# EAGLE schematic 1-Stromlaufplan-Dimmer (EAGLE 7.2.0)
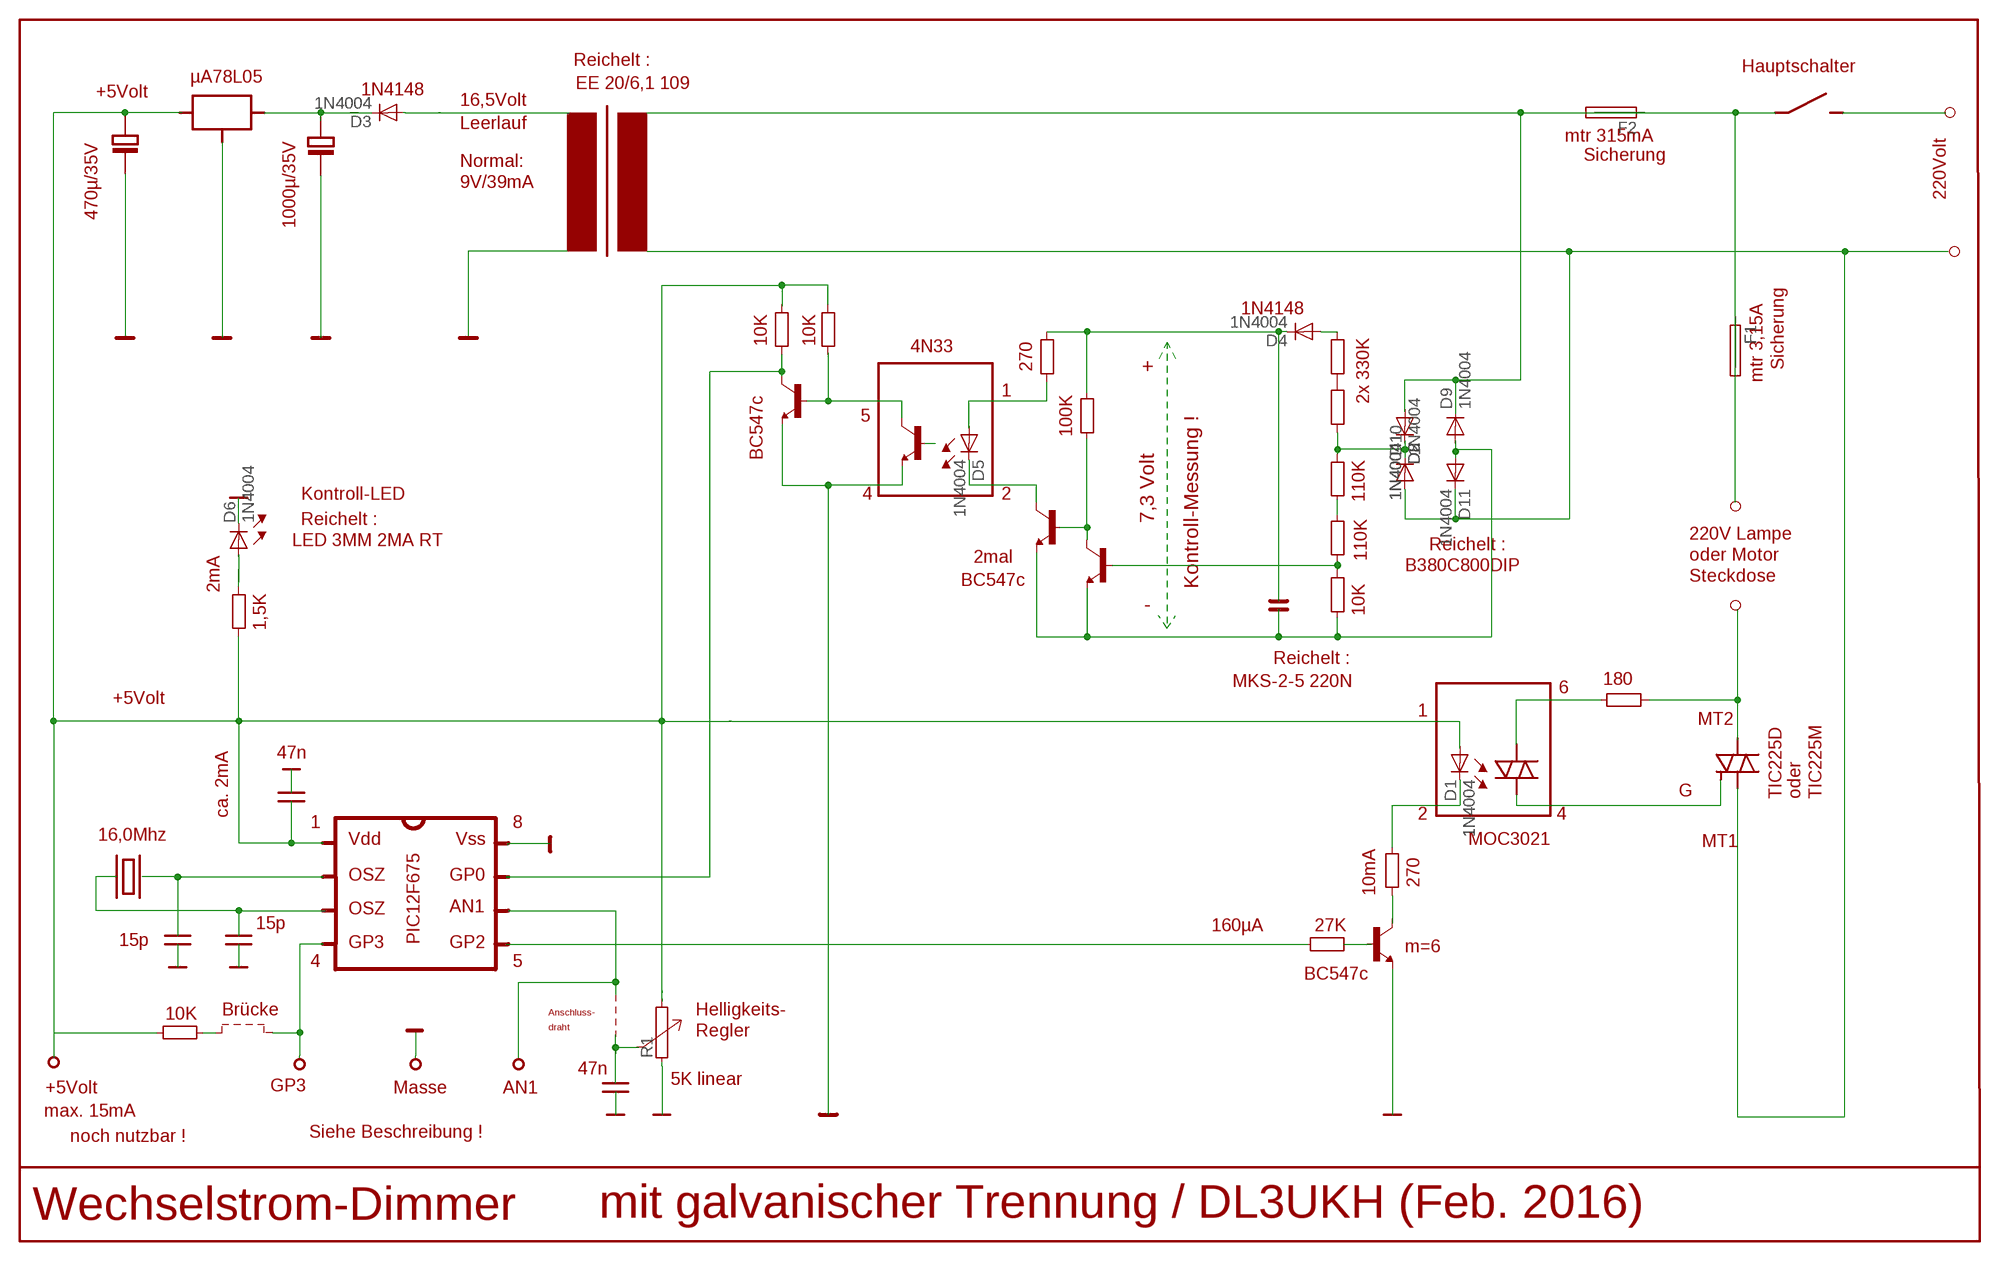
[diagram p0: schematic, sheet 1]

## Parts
D1  1N4004  [DO41-10]
D2  1N4004  [DO41-10]
D3  1N4004  [DO41-10]
D4  1N4004  [DO41-10]
D5  1N4004  [DO41-10]
D6  1N4004  [DO41-10]
D8  1N4004  [DO41-10]
D9  1N4004  [DO41-10]
D10  1N4004  [DO41-10]
D11  1N4004  [DO41-10]
F1  19559  [19559]
F2  19559  [19559]
R1  RHS10  [HS10]

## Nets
N$6: R1.1
N$23: D1.A R1.2
N$27: D1.C
N$28: D2.C D8.C D10.C
N$31: D3.A
N$35: D3.C
N$38: D4.A
N$39: D4.C
N$44: F1.1 F1.2
N$47: D2.A D8.A D9.C F2.1 F2.2
N$49: D9.A D11.A
N$50: D10.A D11.C
N$51: D5.A
N$56: D5.C
N$63: D6.A
N$64: D6.C

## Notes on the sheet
- Reichelt :
- Hauptschalter
- +5Volt | µA78L05
- EE 20/6,1 109
- 1N4148
- 16,5Volt
- Leerlauf
- mtr 315mA | 220Volt
- Sicherung
- Normal:
- 9V/39mA
- 470µ/35V
- 1000µ/35V
- Sicherung
- 1N4148
- 2x 330K
- 10K | 10K
- 4N33
- 270 | +
- mtr 3,15A
- 1
- 5
- 100K
- BC547c
- Kontroll-LED
- 4 | 2 | 110K
- Reichelt :
- 7,3 Volt
- LED 3MM 2MA RT | Reichelt :
- 220V Lampe
- 2mal | 110K | oder Motor
- B380C800DIP
- BC547c | Steckdose
- 2mA | Kontroll-Messung !
- - | 10K
- 1,5K
- Reichelt :
- MKS-2-5 220N | 180
- +5Volt | 6
- 1
- MT2
- 47n
- G | TIC225D | oder | TIC225M
- ca. 2mA | 2 | 4
- 1 | 8
- 16,0Mhz | Vdd | Vss | MOC3021
- MT1
- OSZ | GP0
- 270
- 10mA
- OSZ | AN1
- 15p | 160µA | 27K
- 15p | GP3 | PIC12F675 | GP2
- m=6
- 4 | 5
- BC547c
- 10K | Brücke | Anschluss- | Helligkeits-
- draht
- Regler
- GP3 | 47n
- +5Volt | Masse | AN1 | 5K linear
- max. 15mA
- noch nutzbar ! | Siehe Beschreibung !
- Wechselstrom-Dimmer | mit galvanischer Trennung / DL3UKH (Feb. 2016)

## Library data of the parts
D1-D6 D8-D11 = diode:1N4004: DIODE
F1 F2 = fuse:19559: FUSE HOLDER
R1 = resistor-power:R: Power Resitor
